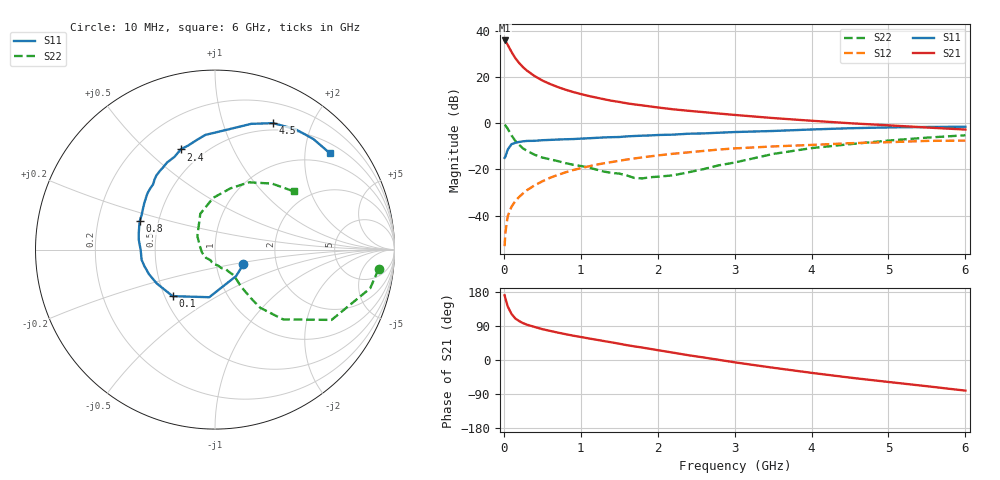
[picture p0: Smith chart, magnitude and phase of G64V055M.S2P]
! SIEMENS Small Signal Semiconductors
! BFG193
! Si NPN RF Bipolar Junction Transistor in SOT223
! VCE = 4 V  IC = 55 mA
! Common Emitter S-Parameters:  August  1996
# GHz  S  MA  R  50
!  f  S11  S21  S12  S22
! GHz  MAG  ANG  MAG  ANG  MAG  ANG  MAG  ANG
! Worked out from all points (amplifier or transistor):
!   36 points, 10 MHz to 6 GHz, reference 50 ohm
!   highest |S21| = 35.7 dB at 10 MHz (marker M1)
!   |S21| within 3 dB of that: start of sweep to 68.24 MHz
!   unconditionally stable (mu >= 1): 390.4 MHz to 2.355 GHz
!   at 250 MHz: K = 0.93, MSG = 27.2 dB, |S12| = -30.3 dB
!   at 1.4 GHz: K = 1.04, MAG = 12.0 dB, |S12| = -16.8 dB
!   at 6 GHz: K = 0.89, MSG = 2.4 dB, |S12| = -7.6 dB
!   S11 on the Smith chart (normalised r, x): 10 MHz: 1.35, -0.23; 100 MHz: 0.55, -0.33; 800 MHz: 0.39, +0.16; 2.4 GHz: 0.38, +0.65; 4.5 GHz: 0.42, +1.48; 6 GHz: 0.73, +2.58
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0.01  0.1779 -27.5  60.98 170.8  0.0022 88.1  0.9178 -6.8
0.02  0.1887 -51.4  58.78 162.8  0.0043 79.5  0.8911 -14.0
0.05  0.2672 -96.9  49.15 141.5  0.0097 70.7  0.7585 -31.1
0.1  0.3507 -132.3  34.44 121.5  0.0157 68.8  0.5434 -45.7
0.15  0.3761 -150.2  25.18 109.4  0.0208 67.1  0.4115 -52.1
0.2  0.3925 -159.6  19.8 102.6  0.0256 68.4  0.3377 -53.5
0.25  0.4038 -166.7  16.12 97.2  0.0304 69.2  0.2835 -54.3
0.3  0.4126 -171.9  13.62 93.2  0.0356 70.0  0.2528 -54.8
0.4  0.4144 180.0  10.38 87.2  0.0453 70.0  0.2071 -54.3
0.5  0.4277 172.9  8.337 81.4  0.0553 69.2  0.1805 -53.9
0.6  0.4339 168.3  7.004 76.9  0.0659 68.0  0.1655 -55.1
0.7  0.4416 163.0  6.031 72.4  0.0759 66.6  0.1513 -57.2
0.8  0.4484 159.1  5.271 68.3  0.0863 64.6  0.137 -59.3
0.9  0.4525 154.5  4.705 64.3  0.0967 62.8  0.1264 -60.7
1.1  0.4709 146.9  3.868 57.1  0.1161 59.3  0.1103 -70.5
1.6  0.5175 130.4  2.677 39.1  0.1639 48.5  0.0739 -103.0
2.2  0.5639 113.6  1.989 19.4  0.2177 34.8  0.0745 -168.5
2.4  0.59 108.9  1.846 12.6  0.2339 30.6  0.0867 166.8
3.5  0.6762 83.1  1.286 -20.4  0.3137 3.4  0.2158 112.3
4.5  0.7754 65.3  0.994 -46.5  0.3683 -16.6  0.3511 76.0
5.5  0.8246 48.3  0.804 -69.2  0.413 -40.0  0.4859 49.2
6  0.8356 39.9  0.726 -80.8  0.4188 -53.4  0.5463 36.4
